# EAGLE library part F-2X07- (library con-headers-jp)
FEMALE HEADER
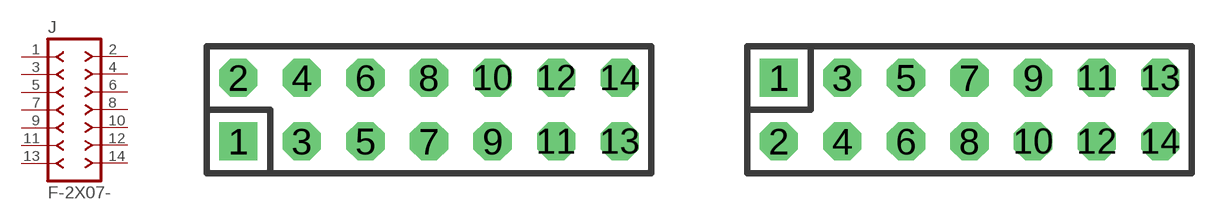
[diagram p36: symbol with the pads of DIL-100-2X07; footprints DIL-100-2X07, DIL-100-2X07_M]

Designator prefix J

## F-2X07-DIL-100  [DIL-100-2X07]
1  1  pas
2  2  pas
3  3  pas
4  4  pas
5  5  pas
6  6  pas
7  7  pas
8  8  pas
9  9  pas
10  10  pas
11  11  pas
12  12  pas
13  13  pas
14  14  pas

## F-2X07-DIL-100_M  [DIL-100-2X07_M]
Pads as for DIL-100-2X07

## F-2X07-DIL-2MM  [DIL-2MM-2X07]
Pads as for DIL-100-2X07

## F-2X07-DIL-2MM_M  [DIL-2MM-2X07_M]
Pads as for DIL-100-2X07

## F-2X07-71991  [71991-14]
Pads as for DIL-100-2X07

## F-2X07-79107  [79107-14]
Pads as for DIL-100-2X07

## F-2X07-79107_M  [79107-14_M]
Pads as for DIL-100-2X07

## Footprint DIL-100-2X07 (pad centres in mm)
PIN HEADER - 0.1"
drill 1.016 square: 1 -7.62,-1.27
drill 1.016 octagon: 2 -7.62,1.27; 3 -5.08,-1.27; 4 -5.08,1.27; 5 -2.54,-1.27; 6 -2.54,1.27; 7 0,-1.27; 8 0,1.27; 9 2.54,-1.27; 10 2.54,1.27; 11 5.08,-1.27; 12 5.08,1.27; 13 7.62,-1.27; 14 7.62,1.27

## Footprint DIL-100-2X07_M (pad centres in mm)
PIN HEADER - MIRRORED 0.1"
drill 1.016 square: 1 -7.62,1.27
drill 1.016 octagon: 2 -7.62,-1.27; 3 -5.08,1.27; 4 -5.08,-1.27; 5 -2.54,1.27; 6 -2.54,-1.27; 7 0,1.27; 8 0,-1.27; 9 2.54,1.27; 10 2.54,-1.27; 11 5.08,1.27; 12 5.08,-1.27; 13 7.62,1.27; 14 7.62,-1.27

## Footprint DIL-2MM-2X07 (pad centres in mm)
PIN HEADER - 2MM"
drill 0.711 square: 1 -6,-1
drill 0.711: 2 -6,1; 3 -4,-1; 4 -4,1; 5 -2,-1; 6 -2,1; 7 0,-1; 8 0,1; 9 2,-1; 10 2,1; 11 4,-1; 12 4,1; 13 6,-1; 14 6,1

## Footprint DIL-2MM-2X07_M (pad centres in mm)
PIN HEADER - MIRRORED 2MM
drill 0.711 square: 1 -6,1
drill 0.711: 2 -6,-1; 3 -4,1; 4 -4,-1; 5 -2,1; 6 -2,-1; 7 0,1; 8 0,-1; 9 2,1; 10 2,-1; 11 4,1; 12 4,-1; 13 6,1; 14 6,-1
